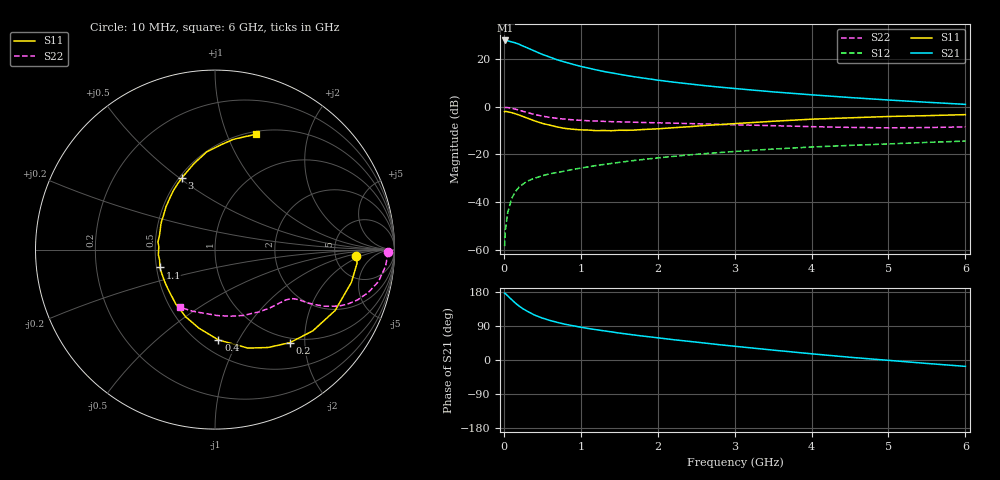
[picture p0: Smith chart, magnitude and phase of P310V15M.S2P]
! SIEMENS Small Signal Semiconductors
! BFP181
! Si NPN RF Bipolar Junction Transistor in SOT143
! VCE = 10 V  IC = 15 mA
! Common Emitter S-Parameters:  March  1996
# GHz  S  MA  R  50
!  f  S11  S21  S12  S22
! GHz  MAG  ANG  MAG  ANG  MAG  ANG  MAG  ANG
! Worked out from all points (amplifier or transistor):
!   36 points, 10 MHz to 6 GHz, reference 50 ohm
!   highest |S21| = 27.7 dB at 20 MHz (marker M1)
!   |S21| within 3 dB of that: start of sweep to 298 MHz
!   unconditionally stable (mu >= 1): 1.158 GHz to end of sweep
!   at 250 MHz: K = 0.39, MSG = 28.9 dB, |S12| = -32.4 dB
!   at 1.4 GHz: K = 1.06, MAG = 17.4 dB, |S12| = -23.8 dB
!   at 6 GHz: K = 1.03, MAG = 6.6 dB, |S12| = -14.4 dB
!   S11 on the Smith chart (normalised r, x): 10 MHz: 8.09, -1.58; 200 MHz: 0.92, -1.70; 400 MHz: 0.61, -0.83; 1.1 GHz: 0.52, -0.12; 3 GHz: 0.52, +0.51; 6 GHz: 0.53, +1.27
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0.01  0.7873 -2.7  24.27 176.3  0.0012 58.8  0.9624 -0.7
0.02  0.7951 -5.5  24.3 175.2  0.0026 75.1  0.9614 -2.1
0.05  0.7815 -13.5  23.89 169.3  0.006 80.5  0.9548 -5.6
0.1  0.7503 -26.9  22.71 159.7  0.0118 74.3  0.9276 -11.1
0.15  0.7086 -39.7  21.63 150.2  0.0167 69.1  0.8873 -15.6
0.2  0.6654 -51.2  20.21 142.1  0.0208 65.9  0.8428 -19.4
0.25  0.6206 -61.5  18.52 135.0  0.024 61.1  0.7981 -22.4
0.3  0.5787 -71.5  17.15 129.2  0.0274 59.0  0.7564 -24.6
0.4  0.5037 -87.8  14.57 118.5  0.0318 55.5  0.685 -27.4
0.5  0.4464 -101.7  12.41 110.7  0.0358 53.6  0.6326 -28.9
0.6  0.4084 -113.6  10.86 104.4  0.0394 52.5  0.5955 -29.9
0.7  0.3736 -125.8  9.483 99.0  0.042 51.6  0.5667 -30.4
0.9  0.3359 -144.5  7.683 90.3  0.0485 51.4  0.5296 -31.4
1.1  0.323 -162.1  6.408 83.0  0.055 51.2  0.5067 -32.6
1.3  0.3167 -174.9  5.444 77.0  0.0616 51.0  0.4916 -34.4
1.6  0.3193 165.9  4.479 68.5  0.0715 50.3  0.4761 -37.2
2.2  0.3619 139.1  3.267 53.7  0.0908 47.2  0.451 -44.8
3  0.4412 114.6  2.398 36.3  0.1152 41.3  0.4169 -57.4
3.5  0.494 103.6  2.039 26.1  0.1295 37.3  0.3997 -66.6
4.5  0.5838 86.9  1.551 7.2  0.1545 28.9  0.3678 -87.8
5.5  0.6477 75.7  1.236 -9.1  0.1785 21.5  0.3654 -110.1
6  0.6806 70.6  1.116 -16.8  0.1901 17.4  0.3763 -121.7
